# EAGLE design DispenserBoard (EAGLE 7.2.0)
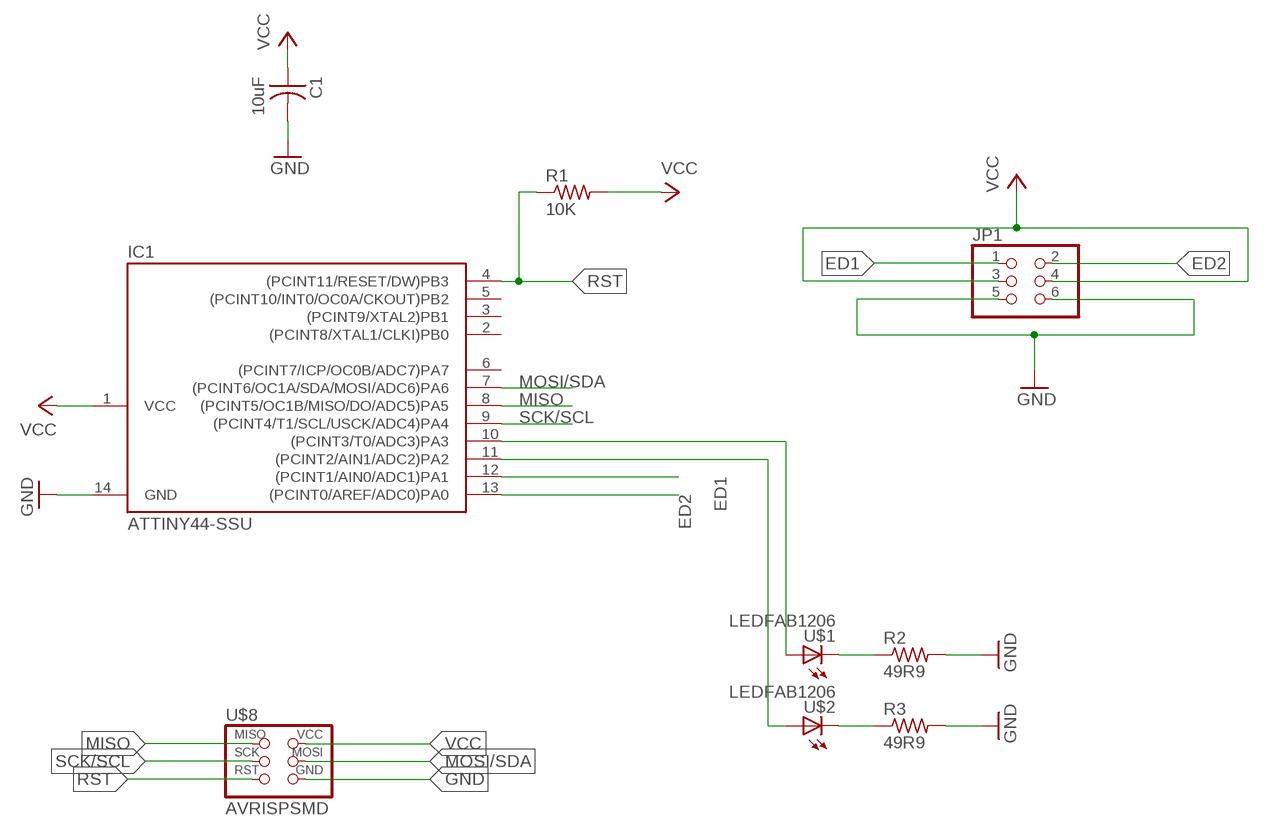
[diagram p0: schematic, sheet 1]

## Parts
C1  10uF  CAP-US1206FAB  [C1206FAB]
IC1  ATTINY44-SSU  [SOIC14]
JP1  PINHD-2X3-SMD  [2X03SMD]
R1  10K  RES-US1206FAB  [R1206FAB]
R2  49R9  RES-US1206FAB  [R1206FAB]
R3  49R9  RES-US1206FAB  [R1206FAB]
U$1  LEDFAB1206  [LED1206FAB]
U$2  LEDFAB1206  [LED1206FAB]
U$8  AVRISPSMD  [2X03SMD]

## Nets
ED1: IC1.12((PCINT1/AIN0/ADC1)PA1) JP1.1
ED2: IC1.13((PCINT0/AREF/ADC0)PA0) JP1.2
GND: C1.2 IC1.14(GND) JP1.5 JP1.6 R2.2 R3.2 U$8.6(GND)
MISO: IC1.8((PCINT5/OC1B/MISO/DO/ADC5)PA5) U$8.1(MISO)
MOSI/SDA: IC1.7((PCINT6/OC1A/SDA/MOSI/ADC6)PA6) U$8.4(MOSI)
N$1: IC1.10((PCINT3/T0/ADC3)PA3) U$1.1(A)
N$2: R2.1 U$1.2(C)
N$3: IC1.11((PCINT2/AIN1/ADC2)PA2) U$2.1(A)
N$4: R3.1 U$2.2(C)
RST: IC1.4((PCINT11/RESET/DW)PB3) R1.1 U$8.5(RST)
SCK/SCL: IC1.9((PCINT4/T1/SCL/USCK/ADC4)PA4) U$8.3(SCK)
VCC: C1.1 IC1.1(VCC) JP1.3 JP1.4 R1.2 U$8.2(VCC)
Unconnected: IC1.2((PCINT8/XTAL1/CLKI)PB0) IC1.3((PCINT9/XTAL2)PB1) IC1.5((PCINT10/INT0/OC0A/CKOUT)PB2) IC1.6((PCINT7/ICP/OC0B/ADC7)PA7)

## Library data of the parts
C1 = fab:CAP-US
IC1 = fab:ATTINY44
JP1 = fab:PINHD-2X3-SMD: PIN HEADER
R1-R3 = fab:RES-US: Resistor (US Symbol)
U$1 U$2 = fab:LED: LED
U$8 = fab:AVRISP

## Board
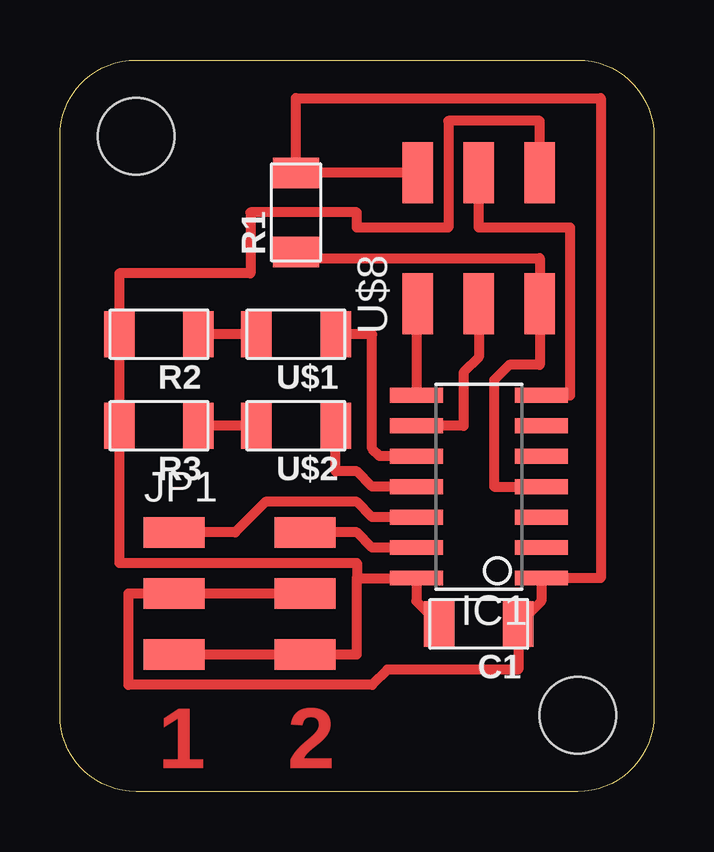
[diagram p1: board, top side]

Size 24.77 x 30.48 mm. Coordinates in mm from the lower left corner, seen from the top.
Outline: 3.17,30.48 21.59,30.48 arc-90 24.77,27.3 24.77,3.17 arc-90 21.59,0 3.17,0 arc-90 0,3.17 0,27.3 arc-90 3.17,30.48
Copper layers (1*16): Top 0.035mm / dielectric 1.5mm / Bottom 0.035mm
Design rules "fabmodule": minimum track width 10mil, minimum drill 0.4mm, track to track 0.42mm, track to pad 0.42mm, pad to pad 0.42mm, via to via 0.42mm, smd to smd 0.42mm, copper to edge 40mil, drill to drill 0.8mm, minimum pad ring 10mil, minimum via ring 8mil, stop-mask expansion 4mil, vias tented up to drill 0mil, thermal gap 10mil
Holes 3.2 mm at 21.59,3.17 3.17,27.3

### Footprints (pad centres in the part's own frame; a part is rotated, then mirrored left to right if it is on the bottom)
C1206FAB = smd 1.27 x 1.905: 1 -1.651,0; 2 1.651,0
SOIC14 = smd 0.61 x 2.21: 1 -3.81,-2.603; 2 -2.54,-2.603; 3 -1.27,-2.603; 4 0,-2.603; 5 1.27,-2.603; 6 2.54,-2.603; 7 3.81,-2.603; 8 3.81,2.603; 9 2.54,2.603; 10 1.27,2.603; 11 0,2.603; 12 -1.27,2.603; 13 -2.54,2.603; 14 -3.81,2.603
2X03SMD = smd 2.54 x 1.27: 1 -2.54,2.54; 2 2.92,2.54; 3 -2.54,0; 4 2.92,0; 5 -2.54,-2.54; 6 2.92,-2.54
R1206FAB = smd 1.27 x 1.905: 1 -1.651,0; 2 1.651,0
LED1206FAB = smd 1.27 x 1.905: 1 -1.651,0; 2 1.651,0

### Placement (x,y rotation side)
C1  17.46,6.99 180 top
IC1  17.46,12.7 90 top
JP1  7.3,8.26 0 top
R1  9.84,24.13 90 top
R2  4.13,19.05 180 top
R3  4.13,15.24 180 top
U$1  9.84,19.05 180 top
U$2  9.84,15.24 180 top
U$8  17.46,22.86 90 top

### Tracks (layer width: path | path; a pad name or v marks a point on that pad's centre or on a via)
ED1
  Top 0.406: IC1.12 13.02,11.43 12.38,12.06 8.57,12.06 7.3,10.79 JP1.1
ED2
  Top 0.406: IC1.13 13.02,10.16 12.38,10.79 JP1.2
GND
  Top 0.406: C1.2 14.86,7.94 IC1.14 12.38,8.89 | JP1.5 JP1.6 12.38,5.71 12.38,8.89 | 12.38,8.89 12.38,9.53 2.48,9.53 R3.2 R2.2 2.48,21.59 7.94,21.59 7.94,24.13 12.38,24.13 12.38,23.5 16.19,23.5 16.19,27.94 20,27.94 U$8.6
MISO
  Top 0.406: U$8.1 14.86,20.32 IC1.8
MOSI/SDA
  Top 0.406: IC1.7 21.27,16.51 21.27,23.5 17.46,23.5 U$8.4
N$1
  Top 0.406: IC1.10 13.34,13.97 13.02,14.29 13.02,19.05 U$1.1
N$2
  Top 0.406: U$1.2 R2.1
N$3
  Top 0.406: IC1.11 13.02,12.7 12.38,13.34 11.49,13.34 U$2.1
N$4
  Top 0.406: U$2.2 R3.1
RST
  Top 0.406: R1.1 10.1,22.23 20,22.23 U$8.5 20,17.78 18.73,17.78 18.1,17.14 18.1,12.7 IC1.4
SCK/SCL
  Top 0.406: U$8.3 17.46,18.1 16.83,17.46 16.83,15.24 IC1.9
VCC
  Top 0.406: U$8.2 R1.2 9.84,28.89 22.54,28.89 22.54,8.89 IC1.1 20.07,7.94 C1.1 19.11,5.08 13.65,5.08 13.02,4.45 2.86,4.45 2.86,8.26 JP1.3 JP1.4

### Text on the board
Top: 1 | 2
